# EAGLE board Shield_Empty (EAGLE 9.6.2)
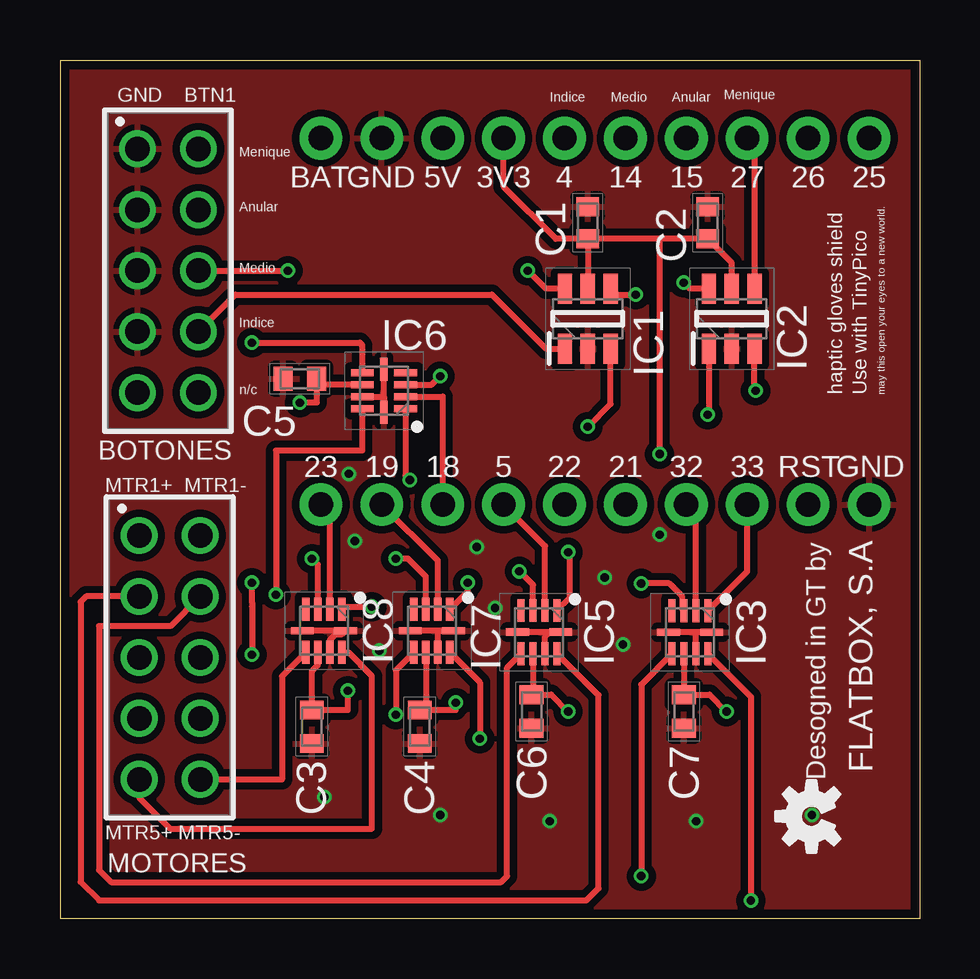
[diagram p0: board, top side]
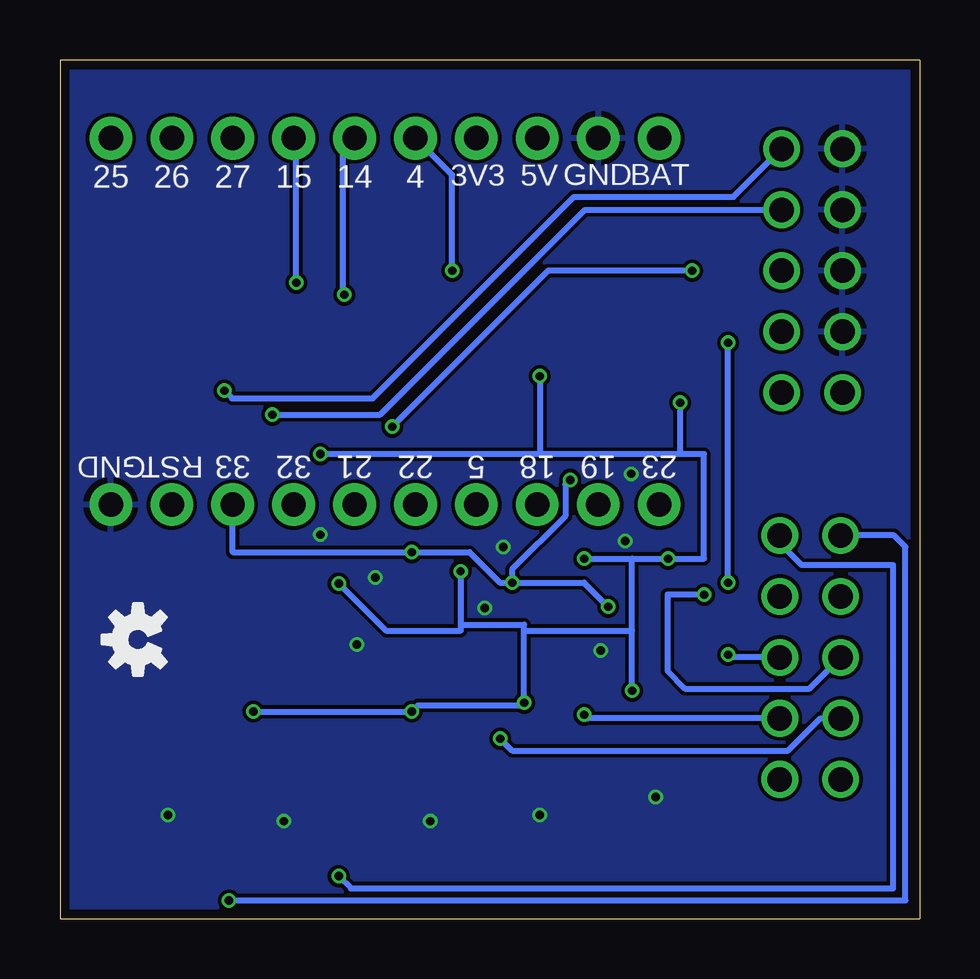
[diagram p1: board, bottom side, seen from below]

Size 35.85 x 35.78 mm. Coordinates in mm from the lower left corner, seen from the top.
Outline: 35.85,0 0,0 0,35.78 35.85,35.78 35.85,0
Copper layers (1*16): Top 0.035559375mm / dielectric 1.6mm / Bottom 0.035559375mm
Design rules "oshpark-2layer": minimum track width 6mil, minimum drill 10mil, track to track 6mil, track to pad 6mil, pad to pad 6mil, via to via 6mil, smd to smd 6mil, copper to edge 15mil, drill to drill 6mil, minimum pad ring 5mil, minimum via ring 5mil, stop-mask expansion 2.5mil, vias tented up to drill 0mil, thermal gap 10mil

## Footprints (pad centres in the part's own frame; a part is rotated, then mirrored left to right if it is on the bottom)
61301021821 = drill 1.02: 1 -5.08,-1.27; 2 -5.08,1.27; 3 -2.54,-1.27; 4 -2.54,1.27; 5 0,-1.27; 6 0,1.27; 7 2.54,-1.27; 8 2.54,1.27; 9 5.08,-1.27; 10 5.08,1.27
CAPC1608X87N = smd 0.8 x 0.94: 1 -0.67,0; 2 0.67,0
CAPC1608X90N = smd 0.78 x 0.99: 1 -0.7,0; 2 0.7,0
SOT95P280X145-6N = smd 1.25 x 0.6: 1 -1.25,0.95; 2 -1.25,0; 3 -1.25,-0.95; 4 1.25,-0.95; 5 1.25,0; 6 1.25,0.95
QFN50P200X200X80-10N = smd 0.95 x 0.3: 1 -0.9,0.75; 2 -0.9,0.25; 3 -0.9,-0.25; 4 -0.9,-0.75; 6 0.9,-0.75; 7 0.9,-0.25; 8 0.9,0.25; 9 0.9,0.75 | smd 0.3 x 0.95: 5 0,-0.9; 10 0,0.9
1X10_NO_SILK = drill 1.016 pad 1.778: 1 0,0; 2 2.54,0; 3 5.08,0; 4 7.62,0; 5 10.16,0; 6 12.7,0; 7 15.24,0; 8 17.78,0; 9 20.32,0; 10 22.86,0

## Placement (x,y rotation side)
BOTONES  BTN 10 PIN  [61301021821]  4.5,27 270 top
C1  0603B104K160CT  [CAPC1608X87N]  22,29 90 top
C2  0603B104K160CT  [CAPC1608X87N]  27,29 90 top
C3  06031C104KAT2A  [CAPC1608X90N]  10.5,8 270 top
C4  06031C104KAT2A  [CAPC1608X90N]  15,8 270 top
C5  06031C104KAT2A  [CAPC1608X90N]  10,22.5 180 top
C6  06031C104KAT2A  [CAPC1608X90N]  19.66,8.63 270 top
C7  06031C104KAT2A  [CAPC1608X90N]  26.01,8.63 270 top
IC1  MAX6817EUT+T  [SOT95P280X145-6N]  22,25 90 top
IC2  MAX6817EUT+T  [SOT95P280X145-6N]  28,25 90 top
IC3  DRV2603RUNR  [QFN50P200X200X80-10N]  26.26,11.94 270 top
IC5  DRV2603RUNR  [QFN50P200X200X80-10N]  19.97,11.94 270 top
IC6  DRV2603RUNR  [QFN50P200X200X80-10N]  13.5,22 180 top
IC7  DRV2603RUNR  [QFN50P200X200X80-10N]  15.5,12 270 top
IC8  DRV2603RUNR  [QFN50P200X200X80-10N]  11,12 270 top
LEFT  [1X10_NO_SILK]  10.87,32.52 0 top
LOGO1  OSHW-LOGOS  [OSHW-LOGO-S]  31.33,4.27 90 top
LOGO2  OSHW-LOGOS  [OSHW-LOGO-S]  32.6,11.63 90 bottom
MOTORES  MTR 10 PIN  [61301021821]  4.58,10.89 270 top
RIGHT  [1X10_NO_SILK]  10.87,17.26 0 top

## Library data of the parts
BOTONES MOTORES = Wurth_Connectors_WR-PHD; DATASHEET-URL: https://katalog.we-online.com/em/datasheet/61301021821.pdf; GENDER: Socket Header; IR: 3A; MATES: WR-PHD 2.54mm SMT Dual Pin Header/THT Angled Dual Pin Header/THT Dual Board Stacker/THT Dual Pin Header; PACKAGING: Tray; PART-NUMBER: 61301021821; PINS: 10; ROWS: Dual; TYPE: Straight
C1 C2 = SamacSys_Parts; DESCRIPTION: WALSIN - 0603B104K160CT - CAP, 0.1F, 16V, 10%, X7R, 0603; HEIGHT: 0.87mm; MANUFACTURER_NAME: Walsin Technology Corporation; MANUFACTURER_PART_NUMBER: 0603B104K160CT; MOUSER_PART_NUMBER: 791-0603B104K160CT; MOUSER_PRICE-STOCK: https://www.mouser.com/Search/Refine.aspx?Keyword=791-0603B104K160CT
C3-C7 = SamacSys_Parts; DESCRIPTION: AVX - 06031C104KAT2A - CAP, MLCC, X7R, 0.1UF, 100V, 0603; HEIGHT: 0.9mm; MANUFACTURER_NAME: AVX; MANUFACTURER_PART_NUMBER: 06031C104KAT2A; MOUSER_PART_NUMBER: 581-06031C104KAT2A; MOUSER_PRICE-STOCK: https://www.mouser.co.uk/ProductDetail/AVX/06031C104KAT2A?qs=oF%2FSscNnLpBUv12UcNAw2A%3D%3D
IC1 IC2 = SamacSys_Parts; DESCRIPTION: Supervisory Circuits Dual Switch Debouncer; HEIGHT: 1.45mm; MANUFACTURER_NAME: Maxim Integrated; MANUFACTURER_PART_NUMBER: MAX6817EUT+T; MOUSER_PART_NUMBER: 700-MAX6817EUTT; MOUSER_PRICE-STOCK: https://www.mouser.co.uk/ProductDetail/Maxim-Integrated/MAX6817EUT%2bT?qs=1THa7WoU59HkU%2FfQtsyW%252BA%3D%3D
IC3 IC5-IC8 = SamacSys_Parts; DESCRIPTION: Haptic Driver with Auto Resonance Tracking for LRA and Optimized Drive for ERM; HEIGHT: 0.8mm; MANUFACTURER_NAME: Texas Instruments; MANUFACTURER_PART_NUMBER: DRV2603RUNR; MOUSER_PART_NUMBER: 595-DRV2603RUNR; MOUSER_PRICE-STOCK: https://www.mouser.co.uk/ProductDetail/Texas-Instruments/DRV2603RUNR?qs=l6ZoeTYLMwNhoGl8Q31%2FaA%3D%3D
LEFT RIGHT = UnexpectedMaker; PROD_ID: CONN-11563
LOGO1 LOGO2 = SparkFun-Aesthetics

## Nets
3.3V: C1.1 C2.1 C3.1 C4.1 C5.1 C6.1 C7.1 IC1.5 IC2.5 IC3.3 IC3.7 IC5.3 IC5.7 IC6.3 IC6.7 IC7.3 IC7.7 IC8.3 IC8.7 LEFT.4
GND: BOTONES.1 BOTONES.3 BOTONES.5 BOTONES.7 C1.2 C2.2 C3.2 C4.2 C5.2 C6.2 C7.2 IC1.2 IC2.2 IC3.5 IC3.8 IC3.10 IC5.5 IC5.8 IC5.10 IC6.5 IC6.8 IC6.10 IC7.5 IC7.8 IC7.10 IC8.5 IC8.8 IC8.10 LEFT.2 RIGHT.10
GPIO4: IC1.6 LEFT.5
GPIO5: IC5.2 RIGHT.4
GPIO14: IC1.4 LEFT.6
GPIO15: IC2.6 LEFT.7
GPIO18: IC6.2 RIGHT.3
GPIO19: IC7.2 RIGHT.2
GPIO21: RIGHT.6
GPIO22: RIGHT.5
GPIO23: IC8.2 RIGHT.1
GPIO25: LEFT.10
GPIO26: LEFT.9
GPIO27: IC2.4 LEFT.8
GPIO32: IC3.2 RIGHT.7
GPIO33: IC3.1 IC5.1 IC6.1 IC7.1 IC8.1 RIGHT.8
MTR1+: IC3.9 MOTORES.1
MTR1-: IC3.6 MOTORES.2
MTR2+: IC5.9 MOTORES.3
MTR2-: IC5.6 MOTORES.4
MTR3+: IC6.9 MOTORES.5
MTR3-: IC6.6 MOTORES.6
MTR4+: IC7.9 MOTORES.7
MTR4-: IC7.6 MOTORES.8
MTR5+: IC8.9 MOTORES.9
MTR5-: IC8.6 MOTORES.10
RESET: RIGHT.9
SW_PUSH_ANULAR: BOTONES.4 IC2.1
SW_PUSH_INDICE: BOTONES.8 IC1.1
SW_PUSH_MEDIO: BOTONES.6 IC1.3
SW_PUSH_MENIQUE: BOTONES.2 IC2.3
USB: LEFT.3
VBAT: LEFT.1

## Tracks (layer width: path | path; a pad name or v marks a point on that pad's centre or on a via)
3.3V  (via drill 0.35)
  Top 0.254: C1.1 20.67,28.33 18.49,30.51 LEFT.4 | 24.99,28.33 C1.1 | C1.1 IC1.5 | IC8.7 10.75,10.58 10.5,10.33 C3.1 12,8.7 v12,9.5 | IC8.3 10.75,14.75 v10.5,15 | IC7.3 15.25,14.25 14.5,15 v14,15 | IC7.7 15.25,8.95 C4.1 16.5,8.7 v16.5,9 | IC6.7 10.7,22.25 C5.1 10.7,21.5 v10,21.5 | IC6.3 15.5,22.25 v15.85,22.6 | IC5.3 19.72,13.91 v19.15,14.48 | IC5.7 19.72,9.4 C6.1 20.48,9.33 v21.18,8.63 | IC3.3 25.94,12.91 25.94,13.43 25.4,13.97 v24.23,13.97 | IC3.7 C7.1 27.09,9.33 v27.79,8.63 | 24.99,28.33 v24.99,19.36 | IC2.5 28,27.33 C2.1 24.99,28.33
  Bottom 0.254: v12,9.5 12,12 | 12,12 12,15 | 12,15 v10.5,15 9,15 9,19.36 10,19.36 | 10,19.36 15.85,19.36 | 15.85,19.36 v24.99,19.36 | v14,15 12,15 | 16.5,12 v16.5,9 16.61,8.89 20.93,8.89 v21.18,8.63 v27.79,8.63 | 16.5,12 16.5,12.25 19.15,12.25 | 16.5,12 12,12 | v10,21.5 10,19.36 | v15.85,22.6 15.85,19.36 | v19.15,14.48 19.15,12.25 | 19.15,12.25 19.15,12 22.26,12 v24.23,13.97
GND  (via drill 0.35)
  Top 0.254: IC8.8 11.25,11.62 11.48,11.85 11.75,11.85 IC8.10 IC8.5 | IC7.8 15.75,12 IC7.10 IC7.5 | IC6.8 13.5,21.75 IC6.10 IC6.5 | IC5.10 20.42,11.94 | 20.42,11.94 IC5.5 | IC5.8 20.22,11.74 20.42,11.94 | IC3.10 26.52,11.94 | 26.52,11.94 IC3.5 | IC3.8 26.51,11.93 26.52,11.94
  other vias: 20.42,4.06 15.85,4.32 11.02,5.08 17.37,15.49 13.31,11.17 18.14,12.95 26.52,4.06 23.47,11.43 22.71,14.22 24.99,16 31.34,4.32 12.29,15.75 12.04,18.54
  pour Top (isolate 0.305): -1.35,37.1 -1.35,-1.33 35.67,-1.33 35.67,37.1
  pour Bottom: 35.89,36.41 35.89,-0.64 -0.77,-0.64 -0.77,36.41
GPIO4  (via drill 0.35)
  Top 0.254: IC1.6 20.25,26.25 v19.5,27
  Bottom 0.254: v19.5,27 19.5,30.99 LEFT.5
GPIO5
  Top 0.254: IC5.2 20.22,15.53 RIGHT.4
GPIO14  (via drill 0.35)
  Top 0.254: IC1.4 23.2,26 v24,26
  Bottom 0.254: LEFT.6 24.07,32.02 24.07,26.07 v24,26
GPIO15  (via drill 0.35)
  Top 0.254: IC2.6 26.25,26.25 v26,26.5
  Bottom 0.254: v26,26.5 26,32.41 LEFT.7
GPIO18
  Top 0.254: IC6.2 15.95,21.75 RIGHT.3
GPIO19
  Top 0.254: IC7.2 15.75,14.92 RIGHT.2
GPIO23
  Top 0.254: IC8.2 11.25,16.88 RIGHT.1
GPIO27
  Top 0.254: IC2.4 28.95,32.22 LEFT.8
GPIO32
  Top 0.254: IC3.2 26.51,16.86 RIGHT.7
GPIO33  (via drill 0.35)
  Top 0.254: IC8.1 11.85,13 v13,13 | IC7.1 17,13.65 v17,14 | IC6.1 14.4,18.47 v14.58,18.29 | IC5.1 21.23,13.35 21.23,15.22 v21.18,15.27 | IC3.1 28.65,14.47 RIGHT.8
  Bottom 0.254: v17,14 17.51,14 18.78,15.27 v21.18,15.27 28.65,15.27 RIGHT.8 | v17,14 14,14 v13,13 | v14.58,18.29 14.78,18.08 14.78,16.77 17,14.56 v17,14
MTR1+  (via drill 0.35)
  Top 0.254: IC3.9 28.8,9.25 v28.8,0.76
  Bottom 0.254: v28.8,0.76 0.61,0.76 0.61,15.49 1.09,15.97 MOTORES.1
MTR1-  (via drill 0.35)
  Top 0.254: IC3.6 24.23,9.75 v24.23,1.78
  Bottom 0.254: v24.23,1.78 23.72,1.27 1.12,1.27 1.12,14.73 4.93,14.73 5.85,15.65 MOTORES.2
MTR2+
  Top 0.254: MOTORES.3 1.09,13.43 0.86,13.21 0.86,1.52 1.63,0.76 21.95,0.76 22.45,1.27 22.45,9.31 IC5.9
MTR2-
  Top 0.254: MOTORES.4 4.61,12.19 1.63,12.19 1.63,2.03 2.13,1.52 18.39,1.52 18.64,1.78 18.64,10.47 IC5.6
MTR3+  (via drill 0.35)
  Top 0.254: IC6.9 12.6,19.5 9,19.5 v9,13.5
  Bottom 0.254: v9,13.5 10.52,13.5 10.52,10.32 9.79,9.59 4.6,9.59 MOTORES.5
MTR3-  (via drill 0.35)
  Top 0.254: v8,11 8,13 8,13.18 v8,14 | v8,24 12.5,24 12.6,23.9 IC6.6
  Bottom 0.254: MOTORES.6 7.89,10.89 v8,11 | v8,14 v8,24
MTR4+  (via drill 0.35)
  Top 0.254: IC7.9 17.5,9.85 v17.5,7.5
  Bottom 0.254: v17.5,7.5 17,7 5.5,7 4.15,8.35 MOTORES.7
MTR4-  (via drill 0.35)
  Top 0.254: v14,8.5 14,10.35 IC7.6
  Bottom 0.254: MOTORES.8 13.85,8.35 v14,8.5
MTR5+
  Top 0.254: MOTORES.9 3.3,5.05 4.6,3.75 13,3.75 13,10.1 12.54,10.56 12.54,10.59 12.04,11.1 IC8.9
MTR5-
  Top 0.254: IC8.6 9.25,10.1 9.25,5.81 MOTORES.10
SW_PUSH_ANULAR  (via drill 0.35)
  Top 0.254: IC2.1 27.05,21.05 v27,21
  Bottom 0.254: v27,21 22.5,21 13.96,29.54 BOTONES.4
SW_PUSH_INDICE
  Top 0.254: BOTONES.8 7.31,26 18,26 20.25,23.75 IC1.1
SW_PUSH_MEDIO  (via drill 0.35)
  Top 0.254: BOTONES.6 v9.5,27 | v22,20.5 22.95,21.45 IC1.3
  Bottom 0.254: v9.5,27 15.5,27 v22,20.5
SW_PUSH_MENIQUE  (via drill 0.35)
  Top 0.254: v29,22 28.95,22.05 IC2.3
  Bottom 0.254: BOTONES.2 7.77,30.08 14.42,30.08 22.82,21.68 28.68,21.68 v29,22

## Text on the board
tPlace: Menique | GND | BTN1 | Indice | Medio | Anular | Menique | Anular | Medio | Indice | n/c | haptic gloves shield | Use with TinyPico | may this open your eyes to a new world. | MTR1+ | MTR1- | Desogned in GT by | FLATBOX, S.A | MTR5+ | MTR5-
tNames: BAT | GND | 5V | 3V3 | 4 | 14 | 15 | 27 | 26 | 25 | 23 | 19 | 18 | 5 | 22 | 21 | 32 | 33 | RST | GND
bNames: BAT | GND | 5V | 3V3 | 4 | 14 | 15 | 27 | 26 | 25 | RST | GND | 23 | 19 | 18 | 5 | 22 | 21 | 32 | 33

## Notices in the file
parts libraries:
SparkFun-Aesthetics: Licensing: Creative Commons ShareAlike 4.0 International - https://creativecommons.org/licenses/by-sa/4.0
Wurth_Connectors_WR-PHD: Copyright: Würth Elektronik
